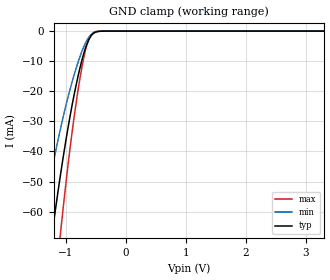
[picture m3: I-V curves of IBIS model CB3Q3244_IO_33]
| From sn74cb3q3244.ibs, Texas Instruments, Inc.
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[Model]   CB3Q3244_IO_33
Model_type  Terminator
| variable   typ   min   max
C_comp   3.08pF   2.85pF   3.89pF
| C_tri-state   3.08pF   2.85pF   3.89pF
[Temperature Range]   40   100   -40
| Ambient temperature   25   85   -40
[Voltage range]   3.3   3   3.6
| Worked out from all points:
|   GND clamp passes 1 mA (typ) near -0.55 V on its own axis
[GND Clamp]
| CB3Q3244_IO_33
|   Voltage   I(typ)   I(min)   I(max)
-5.5V     -958.6mA   -743.8mA   -1.181A
-1.425V   -98.09mA   -66.98mA   -137.7mA
-1.23V    -67.58mA   -45.92mA   -95.43mA
-1.205V   -63.92mA   -43.42mA   -90.26mA
-1.1V     -49.24mA   -33.47mA   -69.33mA
-1.08V    -46.59mA   -31.68mA   -65.51mA
-915mV    -26.72mA   -18.31mA   -36.63mA
-775mV    -13.16mA   -9.118mA   -17mA
-655mV    -4.671mA   -3.306mA   -5.004mA
-550mV    -945.1uA   -723.8uA   -616.3uA
-330mV    -3.342uA   -5.391uA   -293.8nA
3.3V      327.8pA    939.3pA    168.2pA
